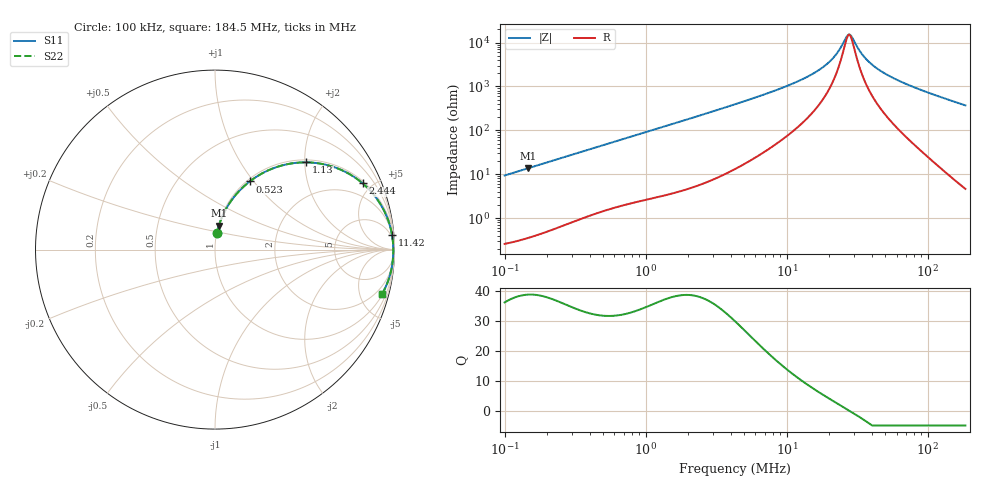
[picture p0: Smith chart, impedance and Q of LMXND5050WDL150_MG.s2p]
! LMXND5050WDL150_MG  S-PARAMETER MODEL  ( General Type )
! Model Generated by TAIYO YUDEN Corporation (http://www.ty-top.com)
! Version 1.0
! TAIYO YUDEN Control No. 191023NI43SB-FBB
! Copyright(c) 2019 TAIYO YUDEN CO.,LTD. All Rights Reserved.
! Product Description (link to TY-COMPAS)
! https://ds.yuden.co.jp/TYCOMPAS/or/detail?pn=LMXND5050WDL150MMG&u=M
! Products Name : Inductors
! Characteristics :
!  Inductance : 15 uH , SRF(min) : 18 MHz , DC Resistance(max) : 0.204 Ohm
!  Rated Current : Saturation :1400 mA , Temp Rise : 1000 mA
!  Case Size : 4.9 x 4.9 / 0.193 x 0.193 [mm/inch] , Thickness : 2.4 / 0.094 [mm/inch]
!  (Conditions: Temperature = 25 degC , DC Bias Current/Voltage = 0A / 0V)
! External Node Assignments :
!  1  o---GGG---o  2
! GND o---------o GND
! Frequency Range : 0.1MHz  -  184.468258MHz  [ 402 STEP ]
# MHz S RI R 50
! Freq[MHz].  S11 Real  S11 Imag  S21 Real  S21 Imag  S12 Real  S12 Imag  S22 Real  S22 Imag
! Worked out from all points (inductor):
!   401 points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, 100 kHz to 184.5 MHz, reference 50 ohm
!   read as one part in series: L = 14.9 uH near 103.8 kHz
!   highest Q = 38.9 at 145.6 kHz (marker M1), where L = 14.9 uH
!   self-resonance near 27.62 MHz
!   S11 on the Smith chart (normalised r, x): 100 kHz: 1.01, +0.19; 523 kHz: 1.03, +0.96; 1.13 MHz: 1.06, +2.04; 2.444 MHz: 1.12, +4.40; 11.42 MHz: 3, +24; 184.5 MHz: 1.09, -7.41
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0.1  0.0112 0.0922  0.9888 -0.0922  0.9888 -0.0922  0.0112 0.0922
0.145645  0.0214 0.1325  0.9786 -0.1325  0.9786 -0.1325  0.0214 0.1325
0.352405  0.1027 0.2889  0.8973 -0.2889  0.8973 -0.2889  0.1027 0.2889
0.523001  0.1938 0.3798  0.8062 -0.3798  0.8062 -0.3798  0.1938 0.3798
1.130472  0.5089 0.4861  0.4911 -0.4861  0.4911 -0.4861  0.5089 0.4861
1.241892  0.5539 0.4836  0.4461 -0.4836  0.4461 -0.4836  0.5539 0.4836
2.443525  0.8223 0.3694  0.1777 -0.3694  0.1777 -0.3694  0.8223 0.3694
4.294977  0.9321 0.2355  0.0679 -0.2355  0.0679 -0.2355  0.9321 0.2355
11.41644  0.9866 0.0799  0.0134 -0.0799  0.0134 -0.0799  0.9866 0.0799
15.13571  0.9906 0.0511  0.00941 -0.0511  0.00941 -0.0511  0.9906 0.0511
18.26631  0.9921 0.0342  0.00787 -0.0342  0.00787 -0.0342  0.9921 0.0342
20.83552  0.9928 0.023  0.00717 -0.023  0.00717 -0.023  0.9928 0.023
23.32347  0.9932 0.0137  0.00677 -0.0137  0.00677 -0.0137  0.9932 0.0137
26.60399  0.9935 0.00312  0.00652 -0.00312  0.00652 -0.00312  0.9935 0.00312
27.62336  0.9935 9.96e-05  0.00649 -9.96e-05  0.00649 -9.96e-05  0.9935 9.96e-05
28.68178  0.9935 -0.00292  0.00647 0.00292  0.00647 0.00292  0.9935 -0.00292
33.33684  0.9934 -0.0151  0.00659 0.0151  0.00659 0.0151  0.9934 -0.0151
37.31757  0.9931 -0.0244  0.00686 0.0244  0.00686 0.0244  0.9931 -0.0244
43.37423  0.9925 -0.0374  0.00752 0.0374  0.00752 0.0374  0.9925 -0.0374
53.33896  0.9909 -0.0567  0.00908 0.0567  0.00908 0.0567  0.9909 -0.0567
88.61236  0.9814 -0.1159  0.0186 0.1159  0.0186 0.1159  0.9814 -0.1159
184.4683  0.9294 -0.2501  0.0706 0.2501  0.0706 0.2501  0.9294 -0.2501
